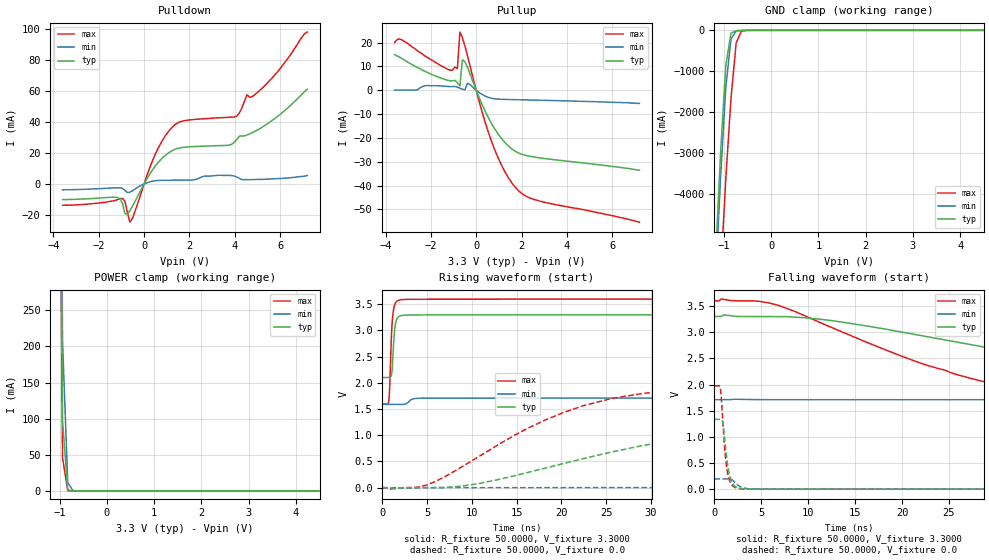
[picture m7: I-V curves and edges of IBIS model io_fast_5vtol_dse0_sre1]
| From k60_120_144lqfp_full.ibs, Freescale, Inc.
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[Model]  io_fast_5vtol_dse0_sre1
|   Model io_fast_5vtol_dse0_sre1
| Library cells for typ/min/max conditions are connected as defined below:
|  pad - External Pad
|  ipp_do - Core Input
|  ipp_obe - Output Buffer Enable
|  esd_boost - vdd_s_3v
|  esd_bus - vdd_s_3v
|  ipp_ame - vss_s_lv
|  ipp_dse - vss_s_lv
|  ipp_ina40a_5vtol - NC
|  ipp_ina40b_5vtol - NC
|  ipp_ina_5vtol - NC
|  ipp_ina_mux_3v - NC
|  ipp_ind - NC
|  ipp_ind_3v - NC
|  ipp_pue - vss_s_lv
|  ipp_sre - vdd_s_lv
|  tie_3v - vdd_s_3v
|  tie_hi - vdd_s_lv
|  vbuf_3v - vdd_s_3v
|  vdd_bulk_lv - vdd_s_lv
|  vdd_s_3v - vdd_s_3v
|  vdd_s_lv - vdd_s_lv
|  vss_bulk - vss_s_3v
|  vss_s_3v - vss_s_3v
|  vss_s_lv - vss_s_lv
| All other pins connected to ground
Model_type I/O
Polarity   Non-Inverting
Enable   Active-High
Vinl =   1.1550V
Vinh =   2.3100V
Vmeas =  1.6500V
Cref =   25.0000pF
Rref =   50.0000
Vref =   0.0V
C_comp   4.6080pF   4.5393pF   4.8314pF
[Temperature Range]   25.0000   0.1250k   -40.0000
[Voltage Range]   3.3000V   1.7100V   3.6000V
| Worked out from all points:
|   slope of the pulldown table from 0 to 0.495 V, typ, clamps not added: 43 ohm
|   slope of the pullup table from 0 to 0.495 V, typ, clamps not added: 46.1 ohm
|   GND clamp passes 1 mA (typ) near -0.54 V on its own axis
|   POWER clamp passes 1 mA (typ) near -0.79 V on its own axis
|   rising waveform, R_fixture 50.0000, V_fixture 3.3000: 20-80 % time 278ps typ, 523ps min, 278ps max; typ from 2.1 V to 3.3 V
|   rising waveform, R_fixture 50.0000, V_fixture 0.0: 20-80 % time 24.1ns typ, 68.1ns min, 14ns max; typ from 0 V to 1.33 V
|   falling waveform, R_fixture 50.0000, V_fixture 3.3000: 20-80 % time 27.2ns typ, 72.5ns min, 19.1ns max; typ from 3.3 V to 2.1 V
|   falling waveform, R_fixture 50.0000, V_fixture 0.0: 20-80 % time 572ps typ, 811ps min, 522ps max; typ from 1.33 V to 0 V
[Pulldown]
|Voltage   I(typ)   I(min)   I(max)
-3.6V     -10.1mA    -3.79mA    -13.73mA
-1.29V    -8.593mA   -2.576mA   -10.67mA
-960mV    -12.21mA   -2.816mA   -9.278mA
-850mV    -18.97mA   -4.143mA   -11mA
-630mV    -17.18mA   -5.368mA   -24.63mA
470mV     11.04mA    1.994mA    18.36mA
1.24V     21.41mA    2.381mA    36.48mA
4.1V      28.81mA    4.4mA      43.8mA
4.54V     31.46mA    2.7mA      57.37mA
4.76V     32.88mA    2.8mA      56.16mA
5.64V     40.8mA     3.2mA      68mA
7.2V      60.9mA     5.4mA      97.7mA
[Pullup]
|Voltage   I(typ)   I(min)   I(max)
-3.6V     15mA       100uA      20.1mA
-3.25V    13.2mA     100uA      21mA
-1.05V    3.94mA     1.56mA     8.456mA
-830mV    3.101mA    1.332mA    9.14mA
-720mV    1.84mA     871.3uA    24.43mA
-610mV    12.78mA    468.4uA    22.17mA
-500mV    12.05mA    179.4uA    18.59mA
-390mV    9.861mA    2.869mA    14.67mA
710mV     -14.5mA    -3.437mA   -22.29mA
1.81V     -26.05mA   -3.957mA   -41.62mA
2.8V      -28.38mA   -4.174mA   -46.51mA
7.2V      -33.58mA   -5.5mA     -55.39mA
[GND_clamp]
|Voltage   I(typ)   I(min)   I(max)
-3.6V     -73.34A    -73.38A    -74.77A
-1.18V    -5.66A     -6.204A    -8.642A
-1.07V    -2.998A    -3.591A    -5.955A
-960mV    -859.3mA   -1.396A    -3.637A
-850mV    -67.61mA   -209.6mA   -1.663A
-740mV    -7.668mA   -15.82mA   -304.8mA
-630mV    -2.587mA   -2.146mA   -18.83mA
-520mV    -662.1uA   -523uA     -1.741mA
7.2V      0A         0A         0A
[POWER_clamp]
|Voltage   I(typ)   I(min)   I(max)
-3.6V     45.85A     45.45A     46.17A
-1.05V    1.004A     1.14A      941.6mA
-940mV    96.57mA    206.1mA    45.73mA
-830mV    1.646mA    11.48mA    218.1uA
-720mV    22.84uA    474.3uA    919.1nA
-610mV    316.6nA    19.24uA    4.178nA
7.2V      0A         0A         0A
[Ramp]
| variable   typ   min   max
dV/dt_r  0.8012/24.0524n   0.1153/68.0945n   1.1861/13.9678n
dV/dt_f  0.7188/27.2464n   69.2148m/72.4012n   1.2016/19.1270n
R_load = 50.0000
[Rising Waveform]
R_fixture= 50.0000
V_fixture= 3.3000
V_fixture_min= 1.7100
V_fixture_max= 3.6000
|time   V(typ)   V(min)   V(max)
0s        2.102V     1.589V     1.597V
731.6ps   2.103V     1.589V     1.669V
802ps     2.103V     1.589V     1.848V
1.066ns   2.206V     1.589V     3.081V
1.26ns    2.772V     1.589V     3.415V
1.383ns   3.033V     1.589V     3.494V
1.614ns   3.218V     1.59V      3.557V
2.344ns   3.291V     1.59V      3.592V
5.445ns   3.298V     1.709V     3.597V
250ns     3.3V       1.71V      3.6V
[Rising Waveform]
R_fixture= 50.0000
V_fixture= 0.0
V_fixture_min= 0.0
V_fixture_max= 0.0
|time   V(typ)   V(min)   V(max)
0s        1.032nV    107.1nV    632.6pV
3.849ns   -568.3uV   -1.899mV   8.023mV
5.922ns   1.102mV    -70.43uV   117mV
16.39ns   296.4mV    -77.45uV   1.147V
22.46ns   554.7mV    -77.38uV   1.565V
29.22ns   807.4mV    -15.11uV   1.802V
37.72ns   1.028V     1.017mV    1.913V
49.02ns   1.2V       6.042mV    1.959V
74.44ns   1.314V     40.75mV    1.976V
250ns     1.335V     192.1mV    1.977V
[Falling Waveform]
R_fixture= 50.0000
V_fixture= 3.3000
V_fixture_min= 1.7100
V_fixture_max= 3.6000
|time   V(typ)   V(min)   V(max)
0s        3.3V       1.71V      3.6V
4.035ns   3.3V       1.713V     3.6V
6.92ns    3.299V     1.71V      3.507V
21.28ns   2.961V     1.71V      2.453V
28.06ns   2.739V     1.71V      2.083V
36.08ns   2.505V     1.71V      1.839V
44.45ns   2.354V     1.709V     1.731V
62.23ns   2.21V      1.701V     1.643V
90.73ns   2.134V     1.674V     1.607V
250ns     2.102V     1.595V     1.597V
[Falling Waveform]
R_fixture= 50.0000
V_fixture= 0.0
V_fixture_min= 0.0
V_fixture_max= 0.0
|time   V(typ)   V(min)   V(max)
0s        1.335V     194.5mV    1.977V
632.1ps   1.334V     194.5mV    1.924V
733.6ps   1.335V     194.5mV    1.742V
883.6ps   1.278V     194.5mV    1.315V
1.142ns   876mV      194.3mV    655.6mV
1.353ns   533.5mV    194mV      347.4mV
1.475ns   384.5mV    194.9mV    241.5mV
1.96ns    100.5mV    168.1mV    58.61mV
3.128ns   5.99mV     22.17mV    4.124mV
250ns     39.33nV    3.38uV     8.922nV
